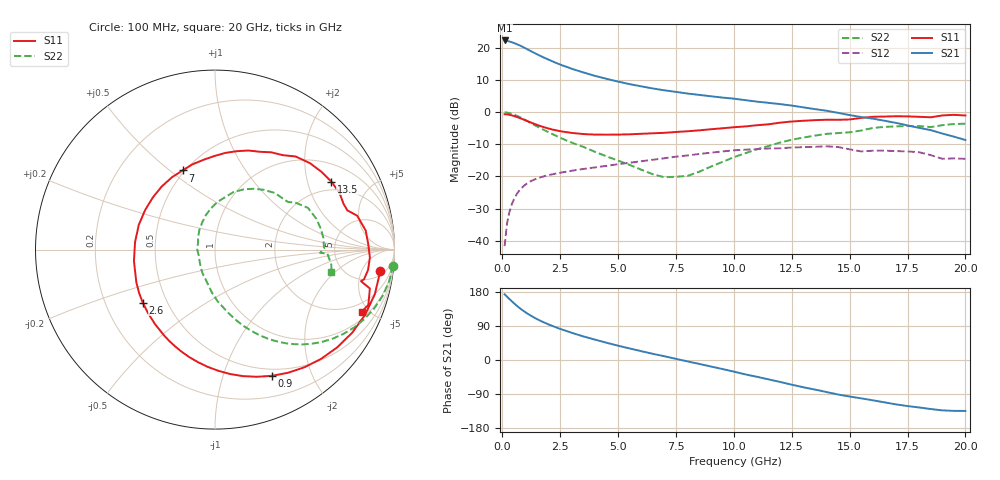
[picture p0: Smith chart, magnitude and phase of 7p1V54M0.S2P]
! Infineon Technologies  Discrete & RF Semiconductors
! bfp620
! VCE =  1.5 V,  IC =  4.0 mA
! Common Emitter S-Parameters:  Sep 2002
# GHz  S  MA  R  50
!  f  S11  S21  S12  S22
! GHz  MAG  ANG  MAG  ANG  MAG  ANG  MAG  ANG
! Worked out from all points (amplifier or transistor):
!   59 points, 100 MHz to 20 GHz, reference 50 ohm
!   highest |S21| = 22.3 dB at 100 MHz (marker M1)
!   |S21| within 3 dB of that: start of sweep to 1.15 GHz
!   unconditionally stable (mu >= 1): 5.112 GHz to 11.85 GHz; 14.62 GHz to 15.45 GHz; 17.16 GHz to end of sweep
!   at 1 GHz: K = 0.27, MSG = 21.2 dB, |S12| = -22.5 dB
!   at 5.5 GHz: K = 1.03, MAG = 11.2 dB, |S12| = -15.8 dB
!   at 20 GHz: K = 1.42, MAG = -0.9 dB, |S12| = -14.5 dB
!   S11 on the Smith chart (normalised r, x): 100 MHz: 7, -12; 900 MHz: 0.42, -1.47; 2.6 GHz: 0.37, -0.29; 7 GHz: 0.49, +0.56; 13.5 GHz: 1.63, +2.84; 20 GHz: 1.38, -4.54
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0.1  0.9286 -7.5  13.07 173.3  0.0082 86.3  0.9948 -5.2
0.2  0.9245 -15.6  12.88 167.4  0.0181 82.0  0.9865 -10.3
0.3  0.9118 -23.5  12.62 161.4  0.0273 77.7  0.9693 -15.4
0.5  0.8722 -38.6  11.94 149.9  0.0439 69.5  0.9182 -24.9
0.7  0.8236 -52.7  11.15 139.5  0.058 62.1  0.8551 -33.4
0.9  0.772 -65.6  10.31 130.2  0.0696 55.6  0.7873 -40.8
1.1  0.7216 -77.6  9.459 122.0  0.0791 50.1  0.7199 -47.2
1.3  0.6752 -88.5  8.665 114.6  0.0867 45.4  0.6568 -52.7
1.5  0.6343 -98.6  7.96 107.9  0.0929 41.5  0.6001 -57.4
1.7  0.5992 -107.9  7.349 101.9  0.098 38.3  0.5503 -61.4
2.2  0.5331 -128.8  6.106 89.0  0.1085 32.2  0.4495 -69.9
2.6  0.4995 -143.7  5.34 80.0  0.1157 28.5  0.3856 -75.6
3  0.4751 -157.2  4.735 71.7  0.1225 25.3  0.335 -80.8
3.5  0.4561 -171.9  4.153 62.3  0.1305 21.8  0.2881 -87.1
5  0.4474 150.4  2.991 37.7  0.1546 12.9  0.1762 -106.8
7  0.4767 112.3  2.188 9.9  0.1916 0.5  0.0971 -158.3
8.5  0.5208 90.6  1.858 -10.3  0.2231 -11.1  0.118 142.8
10.5  0.5998 65.3  1.537 -38.0  0.2606 -30.8  0.2298 95.9
12  0.6863 49.1  1.334 -57.9  0.2739 -44.8  0.3363 72.2
13.5  0.751 30.3  1.115 -78.0  0.2887 -60.2  0.4311 50.5
17  0.8642 -2.9  0.681 -117.1  0.2479 -90.8  0.6009 11.2
20  0.8886 -22.9  0.369 -134.4  0.1876 -106.3  0.6606 -11.1
